| IBIS file stm32h562_563_573_ufbga169.ibs
[IBIS ver] 4.2
[File name] stm32h562_563_573_ufbga169.ibs
[File Rev] 1.1
[Date] 07-05-2024
[Source] Data Created at STMicroelectronics
[Notes]  File originated from ELDO simulations.
[Disclaimer]  This information is for modeling purpose only and is
   not guaranteed. The information is subject to change without
   notice.
[Copyright] Copyright 2024 STMicroelectronics Inc.
|   Component stm32h562_563_573_ufbga169
[Component] stm32h562_563_573_ufbga169
[Manufacturer] STMicroelectronics
[Package]
| variable   typ   min   max
R_pkg  0  NA  NA
L_pkg  0  NA  NA
C_pkg  0  NA  NA
[Pin]   signal_name   model_name
A1  PE2  io8_ft_i3c_spi
A2  PI7  io8_ft_i3c_spi
A3  VDD  power
A4  PB9  io8_ft_i3c_spi
A5  PB6  io8_ft_i3c_spi
A6  PB4  io8_ft_i3c_spi
A7  VDDIO2  power
A8  PG10  io8_ft_i3c_spi
A9  PD3  io8_ft_i3c_spi
A10  VDD  power
A11  PC11  io8_ft_i3c_spi
A12  PA14  io8_ft_i3c_spi
A13  PI2  io8_ft_i3c_spi
B1  PC14-OSC32_IN  io8_ft_i3c_spi
B2  PE3  io8_ft_i3c_spi
B3  VSS  gnd
B4  VCAP  nc
B5  BOOT0  vpphv
B6  PG15  io8_ft_i3c_spi
B7  VSS  gnd
B8  PD7  io8_ft_i3c_spi
B9  PC12  io8_ft_i3c_spi
B10  VSS  gnd
B11  PA15  io8_ft_i3c_spi
B12  PI1  io8_ft_i3c_spi
B13  PI0  io8_ft_i3c_spi
C1  PC15-OSC32_OUT  io8_ft_i3c_spi
C2  PE5  io8_ft_i3c_spi
C3  PI6  io8_ft_i3c_spi
C4  PI4  io8_ft_i3c_spi
C5  PE0  io8_ft_i3c_spi
C6  PB5  io8_ft_i3c_spi
C7  PG14  io8_ft_i3c_spi
C8  PG12  io8_ft_i3c_spi
C9  PD2  io8_ft_i3c_spi
C10  PC10  io8_ft_i3c_spi
C11  PI3  io8_ft_i3c_spi
C12  VSS  gnd
C13  VDD  power
D1  VDD  power
D2  VSS  gnd
D3  PE6  io8_ft_i3c_spi
D4  PE4  io8_ft_i3c_spi
D5  PE1  io8_ft_i3c_spi
D6  PB7  io8_ft_i3c_spi
D7  PG13  io8_ft_i3c_spi
D8  PD5  io8_ft_i3c_spi
D9  PD0  io8_ft_i3c_spi
D10  PH14  io8_ft_i3c_spi
D11  PH15  io8_ft_i3c_spi
D12  PH13  io8_ft_i3c_spi
D13  VDDUSB  power
E1  PF1  io8_ft_i3c_spi
E2  VBAT  power
E3  PI8  io8_ft_i3c_spi
E4  PC13  io8_ft_i3c_spi
E5  PB8  io8_ft_i3c_spi
E6  PB3  io8_ft_i3c_spi
E7  PG11  io8_ft_i3c_spi
E8  PD6  io8_ft_i3c_spi
E9  PD1  io8_ft_i3c_spi
E10  PA10  io8_ft_i3c_spi
E11  PA9  io8_ft_i3c_spi
E12  PA13  io8_ft_i3c_spi
E13  PA12  io8usb_ft_i3c_spi_phy
F1  PF4  io8_ft_i3c_spi
F2  PF2  io8_ft_i3c_spi
F3  PF0  io8_ft_i3c_spi
F4  PI11  io8_ft_i3c_spi
F5  PF3  io8_ft_i3c_spi
F6  PF5  io8_ft_i3c_spi
F7  PG9  io8_ft_i3c_spi
F8  PD4  io8_ft_i3c_spi
F9  PC6  io8_ft_i3c_spi
F10  PC7  io8_ft_i3c_spi
F11  PG8  io8_ft_i3c_spi
F12  PA8  io8_ft_i3c_spi
F13  PA11  io8usb_ft_i3c_spi_phy
G1  VDD  power
G2  VSS  gnd
G3  PF7  io8_ft_i3c_spi
G4  PF6  io8_ft_i3c_spi
G5  PF8  io8_ft_i3c_spi
G6  PF10  io8_ft_i3c_spi
G7  PE8  io8_ft_i3c_spi
G8  PG7  io8_ft_i3c_spi
G9  PG3  io8_ft_i3c_spi
G10  PG5  io8_ft_i3c_spi
G11  PG6  io8_ft_i3c_spi
G12  PC8  io8_ft_i3c_spi
G13  PC9  io8_ft_i3c_spi
H1  PH0-OSC_IN  io8_ft_i3c_spi
H2  PH1-OSC_OUT  io8_ft_i3c_spi
H3  PF9  io8_ft_i3c_spi
H4  NRST  ioreset_ft_v33
H5  PC3  io8_ft_spi
H6  PC5  io8_ft_spi
H7  PF13  io8_ft_spi
H8  PE10  io8_ft_i3c_spi
H9  PD15  io8_ft_i3c_spi
H10  PD11  io8_ft_i3c_spi
H11  PD14  io8_ft_i3c_spi
H12  VSS  gnd
H13  VDD  power
J1  PC0  io8_ft_spi
J2  PC1  io8_ft_spi
J3  PC2  io8_ft_spi
J4  PA0  io8_ft_spi
J5  PA1  io8_ft_spi_tamp
J6  PF11  io8_ft_spi
J7  PF15  io8_ft_i3c_spi
J8  PE14  io8_ft_i3c_spi
J9  PD9  io8_ft_i3c_spi
J10  PB15  io8_ft_spi
J11  PD10  io8_ft_i3c_spi
J12  PG2  io8_ft_i3c_spi
J13  PG4  io8_ft_i3c_spi
K1  VREFM  nc
K2  VSSA  nc
K3  PH2  io8_ft_i3c_spi
K4  PA5  io8_ft_spi
K5  PA7  io8_ft_spi
K6  PB1  io8_ft_spi
K7  PG1  io8_ft_i3c_spi
K8  PE12  io8_ft_i3c_spi
K9  PB10  io8_ft_i3c_spi
K10  PH6  io8_ft_i3c_spi
K11  PB12  io8_ft_i3c_spi
K12  PD12  io8_ft_i3c_spi
K13  PD13  io8_ft_i3c_spi
L1  VDDA  nc
L2  VREFP  nc
L3  PA2  io8_ft_spi
L4  PA4  io8_ft_spi
L5  PB0  io8_ft_spi
L6  PB2  io8_ft_i3c_spi
L7  PG0  io8_ft_i3c_spi
L8  PE9  io8_ft_i3c_spi
L9  PE13  io8_ft_i3c_spi
L10  PH7  io8_ft_i3c_spi
|L11  PB13  io8usb_ft_pd
L11  PB13  nc
L12  PD8  io8_ft_i3c_spi
L13  VDD  power
M1  VDD  power
M2  VSS  gnd
M3  PH5  io8_ft_i3c_spi
M4  VSS  gnd
M5  PA6  io8_ft_spi
M6  PF14  io8_ft_spi
M7  VSS  gnd
M8  PE11  io8_ft_i3c_spi
M9  PB11  io8_ft_i3c_spi
M10  PH8  io8_ft_i3c_spi
M11  PH10  io8_ft_i3c_spi
M12  VSS  gnd
|M13  PB14  io8usb_ft_pd
M13  PB14  nc
N1  PH4  io8_ft_i3c_spi
N2  PH3  io8_ft_i3c_spi
N3  PA3  io8_ft_spi
N4  VDD  power
N5  PC4  io8_ft_spi
N6  PF12  io8_ft_spi
N7  VDD  power
N8  PE7  io8_ft_i3c_spi
N9  PE15  io8_ft_i3c_spi
N10  VCAP  nc
N11  VDD  power
N12  PH11  io8_ft_i3c_spi
N13  PH12  io8_ft_i3c_spi
[Package Model]   484-ufbga-7x7-169-ldo-221014
[Pin Mapping]   pulldown_ref   pullup_ref   | Comment
A1  gndio  vddiom
A2  gndio  vddiom
A3  nc  vddiom
A4  gndio  vddiom  | Depending on IO usage
| A4  gndio  vddmmc  | Depending on IO usage
A5  gndio  vddiom  | Depending on IO usage
| A5  gndio  vddmmc  | Depending on IO usage
A6  gndio  vddiom  | Depending on IO usage
| A6  gndio  vddmmc  | Depending on IO usage
A7  nc  vddmmc
A8  gndio  vddiom  | Depending on IO usage
| A8  gndio  vddmmc  | Depending on IO usage
A9  gndio  vddiom
A10  nc  vddiom
A11  gndio  vddiom
A12  gndio  vddiom
A13  gndio  vddiom
B1  gndio  vddiom  | Depending on IO usage
| B1  gndio  vsw  | Depending on IO usage
B2  gndio  vddiom
B3  gndio  nc
B4  nc  nc
B5  gndio  vddiom  | Depending on IO usage
| B5  gndio  vddmmc  | Depending on IO usage
B6  gndio  vddiom  | Depending on IO usage
| B6  gndio  vddmmc  | Depending on IO usage
B7  gndio  nc
B8  gndio  vddiom  | Depending on IO usage
| B8  gndio  vddmmc  | Depending on IO usage
B9  gndio  vddiom
B10  gndio  nc
B11  gndio  vddiom
B12  gndio  vddiom
B13  gndio  vddiom
C1  gndio  vddiom  | Depending on IO usage
| C1  gndio  vsw  | Depending on IO usage
C2  gndio  vddiom
C3  gndio  vddiom
C4  gndio  vddiom
C5  gndio  vddiom  | Depending on IO usage
| C5  gndio  vddmmc  | Depending on IO usage
C6  gndio  vddiom  | Depending on IO usage
| C6  gndio  vddmmc  | Depending on IO usage
C7  gndio  vddiom  | Depending on IO usage
| C7  gndio  vddmmc  | Depending on IO usage
C8  gndio  vddiom  | Depending on IO usage
| C8  gndio  vddmmc  | Depending on IO usage
C9  gndio  vddiom
C10  gndio  vddiom
C11  gndio  vddiom
C12  gndio  nc
C13  nc  vddiom
D1  nc  vddiom
D2  gndio  nc
D3  gndio  vddiom
D4  gndio  vddiom
D5  gndio  vddiom  | Depending on IO usage
| D5  gndio  vddmmc  | Depending on IO usage
D6  gndio  vddiom  | Depending on IO usage
| D6  gndio  vddmmc  | Depending on IO usage
D7  gndio  vddiom  | Depending on IO usage
| D7  gndio  vddmmc  | Depending on IO usage
D8  gndio  vddiom
D9  gndio  vddiom
D10  gndio  vddiom
D11  gndio  vddiom
D12  gndio  vddiom
D13  nc  vddusb
E1  gndio  vddiom
E2  nc  vsw
E3  gndio  vddiom  | Depending on IO usage
| E3  gndio  vsw  | Depending on IO usage
E4  gndio  vddiom  | Depending on IO usage
| E4  gndio  vsw  | Depending on IO usage
E5  gndio  vddiom  | Depending on IO usage
| E5  gndio  vddmmc  | Depending on IO usage
E6  gndio  vddiom  | Depending on IO usage
| E6  gndio  vddmmc  | Depending on IO usage
E7  gndio  vddiom  | Depending on IO usage
| E7  gndio  vddmmc  | Depending on IO usage
E8  gndio  vddiom  | Depending on IO usage
| E8  gndio  vddmmc  | Depending on IO usage
E9  gndio  vddiom
E10  gndio  vddiom  | Depending on IO usage
| E10  gndio  vddusb  | Depending on IO usage
E11  gndio  vddiom  | Depending on IO usage
| E11  gndio  vddusb  | Depending on IO usage
E12  gndio  vddiom  | Depending on IO usage
| E12  gndio  vddusb  | Depending on IO usage
E13  gndio  vddiom  | Depending on IO usage
| E13  gndio  vddusb  | Depending on IO usage
F1  gndio  vddiom
F2  gndio  vddiom
F3  gndio  vddiom
F4  gndio  vddiom
F5  gndio  vddiom
F6  gndio  vddiom
F7  gndio  vddiom  | Depending on IO usage
| F7  gndio  vddmmc  | Depending on IO usage
F8  gndio  vddiom
F9  gndio  vddiom
F10  gndio  vddiom
F11  gndio  vddiom
F12  gndio  vddiom
F13  gndio  vddiom  | Depending on IO usage
| F13  gndio  vddusb  | Depending on IO usage
G1  nc  vddiom
G2  gndio  nc
G3  gndio  vddiom
G4  gndio  vddiom
G5  gndio  vddiom
G6  gndio  vddiom
G7  gndio  vddiom
G8  gndio  vddiom
G9  gndio  vddiom
G10  gndio  vddiom
G11  gndio  vddiom
G12  gndio  vddiom
G13  gndio  vddiom
H1  gndio  vddiom
H2  gndio  vddiom
H3  gndio  vddiom
H4  gndio  vddiom
H5  gndio  vddiom
H6  gndio  vddiom
H7  gndio  vddiom
H8  gndio  vddiom
H9  gndio  vddiom
H10  gndio  vddiom
H11  gndio  vddiom
H12  gndio  nc
H13  nc  vddiom
J1  gndio  vddiom
J2  gndio  vddiom
J3  gndio  vddiom
J4  gndio  vddiom
J5  gndio  vddiom
J6  gndio  vddiom
J7  gndio  vddiom
J8  gndio  vddiom
J9  gndio  vddiom
J10  gndio  vddiom
J11  gndio  vddiom
J12  gndio  vddiom
J13  gndio  vddiom
K1  nc  nc
K2  nc  nc
K3  gndio  vddiom
K4  gndio  vddiom
K5  gndio  vddiom
K6  gndio  vddiom
K7  gndio  vddiom
K8  gndio  vddiom
K9  gndio  vddiom
K10  gndio  vddiom
K11  gndio  vddiom
K12  gndio  vddiom
K13  gndio  vddiom
L1  nc  nc
L2  nc  nc
L3  gndio  vddiom
L4  gndio  vddiom
L5  gndio  vddiom
L6  gndio  vddiom
L7  gndio  vddiom
L8  gndio  vddiom
L9  gndio  vddiom
L10  gndio  vddiom
|L11  gndio  vddiom
L11  nc nc
L12  gndio  vddiom
L13  nc  vddiom
M1  nc  vddiom
M2  gndio  nc
M3  gndio  vddiom
M4  gndio  nc
M5  gndio  vddiom
M6  gndio  vddiom
M7  gndio  nc
M8  gndio  vddiom
M9  gndio  vddiom
M10  gndio  vddiom
M11  gndio  vddiom
M12  gndio  nc
|M13  gndio  vddiom
M13  nc nc
N1  gndio  vddiom
N2  gndio  vddiom
N3  gndio  vddiom
N4  nc  vddiom
N5  gndio  vddiom
N6  gndio  vddiom
N7  nc  vddiom
N8  gndio  vddiom
N9  gndio  vddiom
N10  nc  nc
N11  nc  vddiom
N12  gndio  vddiom
N13  gndio  vddiom
[Model Selector] io8_ft_i3c_spi
io8_ft_spi_ls_1v2 "io8_ft spi low speed @ 1.2V"
io8_ft_spi_ls_1v8 "io8_ft spi low speed @ 1.8V"
io8_ft_spi_ls_3v3 "io8_ft spi low speed @ 3.3V"
io8_ft_spi_ms_1v2 "io8_ft spi med speed @ 1.2V"
io8_ft_spi_ms_1v8 "io8_ft spi med speed @ 1.8V"
io8_ft_spi_ms_3v3 "io8_ft spi med speed @ 3.3V"
io8_ft_spi_fs_1v2 "io8_ft spi fast speed @ 1.2V"
io8_ft_spi_fs_1v8 "io8_ft spi fast speed @ 1.8V"
io8_ft_spi_fs_3v3 "io8_ft spi fast speed @ 3.3V"
io8_ft_spi_hs_1v2 "io8_ft spi high speed @ 1.2V"
io8_ft_spi_hs_1v8 "io8_ft spi high speed @ 1.8V"
io8_ft_spi_hs_3v3 "io8_ft spi high speed @ 3.3V"
io8_ft_hslv_spi_ls_1v2 "io8_ft spi hslv low speed @ 1.2V"
io8_ft_hslv_spi_ls_1v8 "io8_ft spi hslv low speed @ 1.8V"
io8_ft_hslv_spi_ls_2v5 "io8_ft spi hslv low speed @ 2.5V"
io8_ft_hslv_spi_ms_1v2 "io8_ft spi hslv med speed @ 1.2V"
io8_ft_hslv_spi_ms_1v8 "io8_ft spi hslv med speed @ 1.8V"
io8_ft_hslv_spi_ms_2v5 "io8_ft spi hslv med speed @ 2.5V"
io8_ft_hslv_spi_fs_1v2 "io8_ft spi hslv fast speed @ 1.2V"
io8_ft_hslv_spi_fs_1v8 "io8_ft spi hslv fast speed @ 1.8V"
io8_ft_hslv_spi_fs_2v5 "io8_ft spi hslv fast speed @ 2.5V"
io8_ft_hslv_spi_hs_1v2 "io8_ft spi hslv high speed @ 1.2V"
io8_ft_hslv_spi_hs_1v8 "io8_ft spi hslv high speed @ 1.8V"
io8_ft_hslv_spi_hs_2v5 "io8_ft spi hslv high speed @ 2.5V"
io8_ft_i3c_spi_ls_1v2 "io8_ft i3c spi open-drain low speed @ 1.2V"
io8_ft_i3c_spi_ls_1v8 "io8_ft i3c spi open-drain low speed @ 1.8V"
io8_ft_i3c_spi_ls_3v3 "io8_ft i3c spi open-drain low speed @ 3.3V"
io8_ft_i3c_spi_ms_1v2 "io8_ft i3c spi open-drain med speed @ 1.2V"
io8_ft_i3c_spi_ms_1v8 "io8_ft i3c spi open-drain med speed @ 1.8V"
io8_ft_i3c_spi_ms_3v3 "io8_ft i3c spi open-drain med speed @ 3.3V"
io8_ft_i3c_spi_fs_1v2 "io8_ft i3c spi open-drain fast speed @ 1.2V"
io8_ft_i3c_spi_fs_1v8 "io8_ft i3c spi open-drain fast speed @ 1.8V"
io8_ft_i3c_spi_fs_3v3 "io8_ft i3c spi open-drain fast speed @ 3.3V"
io8_ft_i3c_spi_hs_1v2 "io8_ft i3c spi open-drain high speed @ 1.2V"
io8_ft_i3c_spi_hs_1v8 "io8_ft i3c spi open-drain high speed @ 1.8V"
io8_ft_i3c_spi_hs_3v3 "io8_ft i3c spi open-drain high speed @ 3.3V"
io8_ft_hslv_i3c_spi_ls_1v2 "io8_ft hslv i3c spi open-drain low speed @ 1.2V"
io8_ft_hslv_i3c_spi_ls_1v8 "io8_ft hslv i3c spi open-drain low speed @ 1.8V"
io8_ft_hslv_i3c_spi_ls_2v5 "io8_ft hslv i3c spi open-drain low speed @ 2.5V"
io8_ft_hslv_i3c_spi_ms_1v2 "io8_ft hslv i3c spi open-drain med speed @ 1.2V"
io8_ft_hslv_i3c_spi_ms_1v8 "io8_ft hslv i3c spi open-drain med speed @ 1.8V"
io8_ft_hslv_i3c_spi_ms_2v5 "io8_ft hslv i3c spi open-drain med speed @ 2.5V"
io8_ft_hslv_i3c_spi_fs_1v2 "io8_ft hslv i3c spi open-drain fast speed @ 1.2V"
io8_ft_hslv_i3c_spi_fs_1v8 "io8_ft hslv i3c spi open-drain fast speed @ 1.8V"
io8_ft_hslv_i3c_spi_fs_2v5 "io8_ft hslv i3c spi open-drain fast speed @ 2.5V"
io8_ft_hslv_i3c_spi_hs_1v2 "io8_ft hslv i3c spi open-drain high speed @ 1.2V"
io8_ft_hslv_i3c_spi_hs_1v8 "io8_ft hslv i3c spi open-drain high speed @ 1.8V"
io8_ft_hslv_i3c_spi_hs_2v5 "io8_ft hslv i3c spi open-drain high speed @ 2.5V"
io8_ft_i3c_fmp_spi_3v3 "io8_ft i3c fm+ spi open-drain @ 3.3V"
io8_ft_i3c_fmp_spi_1v8 "io8_ft i3c fm+ spi open-drain @ 1.8V"
io8_ft_i3c_fmp_spi_1v2 "io8_ft i3c fm+ spi open-drain @ 1.2V"
[Model Selector] io8_ft_spi
io8_ft_spi_ls_1v2 "io8_ft spi low speed @ 1.2V"
io8_ft_spi_ls_1v8 "io8_ft spi low speed @ 1.8V"
io8_ft_spi_ls_3v3 "io8_ft spi low speed @ 3.3V"
io8_ft_spi_ms_1v2 "io8_ft spi med speed @ 1.2V"
io8_ft_spi_ms_1v8 "io8_ft spi med speed @ 1.8V"
io8_ft_spi_ms_3v3 "io8_ft spi med speed @ 3.3V"
io8_ft_spi_fs_1v2 "io8_ft spi fast speed @ 1.2V"
io8_ft_spi_fs_1v8 "io8_ft spi fast speed @ 1.8V"
io8_ft_spi_fs_3v3 "io8_ft spi fast speed @ 3.3V"
io8_ft_spi_hs_1v2 "io8_ft spi high speed @ 1.2V"
io8_ft_spi_hs_1v8 "io8_ft spi high speed @ 1.8V"
io8_ft_spi_hs_3v3 "io8_ft spi high speed @ 3.3V"
io8_ft_hslv_spi_ls_1v2 "io8_ft spi hslv low speed @ 1.2V"
io8_ft_hslv_spi_ls_1v8 "io8_ft spi hslv low speed @ 1.8V"
io8_ft_hslv_spi_ls_2v5 "io8_ft spi hslv low speed @ 2.5V"
io8_ft_hslv_spi_ms_1v2 "io8_ft spi hslv med speed @ 1.2V"
io8_ft_hslv_spi_ms_1v8 "io8_ft spi hslv med speed @ 1.8V"
io8_ft_hslv_spi_ms_2v5 "io8_ft spi hslv med speed @ 2.5V"
io8_ft_hslv_spi_fs_1v2 "io8_ft spi hslv fast speed @ 1.2V"
io8_ft_hslv_spi_fs_1v8 "io8_ft spi hslv fast speed @ 1.8V"
io8_ft_hslv_spi_fs_2v5 "io8_ft spi hslv fast speed @ 2.5V"
io8_ft_hslv_spi_hs_1v2 "io8_ft spi hslv high speed @ 1.2V"
io8_ft_hslv_spi_hs_1v8 "io8_ft spi hslv high speed @ 1.8V"
io8_ft_hslv_spi_hs_2v5 "io8_ft spi hslv high speed @ 2.5V"
[Model Selector] io8_ft_spi_tamp
io8_ft_spi_ls_1v2 "io8_ft spi low speed @ 1.2V"
io8_ft_spi_ls_1v8 "io8_ft spi low speed @ 1.8V"
io8_ft_spi_ls_3v3 "io8_ft spi low speed @ 3.3V"
io8_ft_spi_ms_1v2 "io8_ft spi med speed @ 1.2V"
io8_ft_spi_ms_1v8 "io8_ft spi med speed @ 1.8V"
io8_ft_spi_ms_3v3 "io8_ft spi med speed @ 3.3V"
io8_ft_spi_fs_1v2 "io8_ft spi fast speed @ 1.2V"
io8_ft_spi_fs_1v8 "io8_ft spi fast speed @ 1.8V"
io8_ft_spi_fs_3v3 "io8_ft spi fast speed @ 3.3V"
io8_ft_spi_hs_1v2 "io8_ft spi high speed @ 1.2V"
io8_ft_spi_hs_1v8 "io8_ft spi high speed @ 1.8V"
io8_ft_spi_hs_3v3 "io8_ft spi high speed @ 3.3V"
io8_ft_hslv_spi_ls_1v2 "io8_ft spi hslv low speed @ 1.2V"
io8_ft_hslv_spi_ls_1v8 "io8_ft spi hslv low speed @ 1.8V"
io8_ft_hslv_spi_ls_2v5 "io8_ft spi hslv low speed @ 2.5V"
io8_ft_hslv_spi_ms_1v2 "io8_ft spi hslv med speed @ 1.2V"
io8_ft_hslv_spi_ms_1v8 "io8_ft spi hslv med speed @ 1.8V"
io8_ft_hslv_spi_ms_2v5 "io8_ft spi hslv med speed @ 2.5V"
io8_ft_hslv_spi_fs_1v2 "io8_ft spi hslv fast speed @ 1.2V"
io8_ft_hslv_spi_fs_1v8 "io8_ft spi hslv fast speed @ 1.8V"
io8_ft_hslv_spi_fs_2v5 "io8_ft spi hslv fast speed @ 2.5V"
io8_ft_hslv_spi_hs_1v2 "io8_ft spi hslv high speed @ 1.2V"
io8_ft_hslv_spi_hs_1v8 "io8_ft spi hslv high speed @ 1.8V"
io8_ft_hslv_spi_hs_2v5 "io8_ft spi hslv high speed @ 2.5V"
io8_ft_tamp_v33_1v2 "io8_ft tamp V33 @ 1.2V"
io8_ft_tamp_v33_1v8 "io8_ft tamp V33 @ 1.2V"
io8_ft_tamp_v33_3v3 "io8_ft tamp V33 @ 1.2V"
[Model Selector] io8usb_ft_i3c_spi_phy
io8_ft_spi_ls_1v2 "io8_ft spi low speed @ 1.2V"
io8_ft_spi_ls_1v8 "io8_ft spi low speed @ 1.8V"
io8_ft_spi_ls_3v3 "io8_ft spi low speed @ 3.3V"
io8_ft_spi_ms_1v2 "io8_ft spi med speed @ 1.2V"
io8_ft_spi_ms_1v8 "io8_ft spi med speed @ 1.8V"
io8_ft_spi_ms_3v3 "io8_ft spi med speed @ 3.3V"
io8_ft_spi_fs_1v2 "io8_ft spi fast speed @ 1.2V"
io8_ft_spi_fs_1v8 "io8_ft spi fast speed @ 1.8V"
io8_ft_spi_fs_3v3 "io8_ft spi fast speed @ 3.3V"
io8_ft_spi_hs_1v2 "io8_ft spi high speed @ 1.2V"
io8_ft_spi_hs_1v8 "io8_ft spi high speed @ 1.8V"
io8_ft_spi_hs_3v3 "io8_ft spi high speed @ 3.3V"
io8_ft_hslv_spi_ls_1v2 "io8_ft spi hslv low speed @ 1.2V"
io8_ft_hslv_spi_ls_1v8 "io8_ft spi hslv low speed @ 1.8V"
io8_ft_hslv_spi_ls_2v5 "io8_ft spi hslv low speed @ 2.5V"
io8_ft_hslv_spi_ms_1v2 "io8_ft spi hslv med speed @ 1.2V"
io8_ft_hslv_spi_ms_1v8 "io8_ft spi hslv med speed @ 1.8V"
io8_ft_hslv_spi_ms_2v5 "io8_ft spi hslv med speed @ 2.5V"
io8_ft_hslv_spi_fs_1v2 "io8_ft spi hslv fast speed @ 1.2V"
io8_ft_hslv_spi_fs_1v8 "io8_ft spi hslv fast speed @ 1.8V"
io8_ft_hslv_spi_fs_2v5 "io8_ft spi hslv fast speed @ 2.5V"
io8_ft_hslv_spi_hs_1v2 "io8_ft spi hslv high speed @ 1.2V"
io8_ft_hslv_spi_hs_1v8 "io8_ft spi hslv high speed @ 1.8V"
io8_ft_hslv_spi_hs_2v5 "io8_ft spi hslv high speed @ 2.5V"
io8_ft_i3c_spi_ls_1v2 "io8_ft i3c spi open-drain low speed @ 1.2V"
io8_ft_i3c_spi_ls_1v8 "io8_ft i3c spi open-drain low speed @ 1.8V"
io8_ft_i3c_spi_ls_3v3 "io8_ft i3c spi open-drain low speed @ 3.3V"
io8_ft_i3c_spi_ms_1v2 "io8_ft i3c spi open-drain med speed @ 1.2V"
io8_ft_i3c_spi_ms_1v8 "io8_ft i3c spi open-drain med speed @ 1.8V"
io8_ft_i3c_spi_ms_3v3 "io8_ft i3c spi open-drain med speed @ 3.3V"
io8_ft_i3c_spi_fs_1v2 "io8_ft i3c spi open-drain fast speed @ 1.2V"
io8_ft_i3c_spi_fs_1v8 "io8_ft i3c spi open-drain fast speed @ 1.8V"
io8_ft_i3c_spi_fs_3v3 "io8_ft i3c spi open-drain fast speed @ 3.3V"
io8_ft_i3c_spi_hs_1v2 "io8_ft i3c spi open-drain high speed @ 1.2V"
io8_ft_i3c_spi_hs_1v8 "io8_ft i3c spi open-drain high speed @ 1.8V"
io8_ft_i3c_spi_hs_3v3 "io8_ft i3c spi open-drain high speed @ 3.3V"
io8_ft_hslv_i3c_spi_ls_1v2 "io8_ft hslv i3c spi open-drain low speed @ 1.2V"
io8_ft_hslv_i3c_spi_ls_1v8 "io8_ft hslv i3c spi open-drain low speed @ 1.8V"
io8_ft_hslv_i3c_spi_ls_2v5 "io8_ft hslv i3c spi open-drain low speed @ 2.5V"
io8_ft_hslv_i3c_spi_ms_1v2 "io8_ft hslv i3c spi open-drain med speed @ 1.2V"
io8_ft_hslv_i3c_spi_ms_1v8 "io8_ft hslv i3c spi open-drain med speed @ 1.8V"
io8_ft_hslv_i3c_spi_ms_2v5 "io8_ft hslv i3c spi open-drain med speed @ 2.5V"
io8_ft_hslv_i3c_spi_fs_1v2 "io8_ft hslv i3c spi open-drain fast speed @ 1.2V"
io8_ft_hslv_i3c_spi_fs_1v8 "io8_ft hslv i3c spi open-drain fast speed @ 1.8V"
io8_ft_hslv_i3c_spi_fs_2v5 "io8_ft hslv i3c spi open-drain fast speed @ 2.5V"
io8_ft_hslv_i3c_spi_hs_1v2 "io8_ft hslv i3c spi open-drain high speed @ 1.2V"
io8_ft_hslv_i3c_spi_hs_1v8 "io8_ft hslv i3c spi open-drain high speed @ 1.8V"
io8_ft_hslv_i3c_spi_hs_2v5 "io8_ft hslv i3c spi open-drain high speed @ 2.5V"
io8_ft_i3c_fmp_spi_3v3 "io8_ft i3c fm+ spi open-drain @ 3.3V"
io8_ft_i3c_fmp_spi_1v8 "io8_ft i3c fm+ spi open-drain @ 1.8V"
io8_ft_i3c_fmp_spi_1v2 "io8_ft i3c fm+ spi open-drain @ 1.2V"
io8usb_ft_phy_ls_2v5 "iousb ft low speed @ 2.5V"
io8usb_ft_phy_ls_3v3 "iousb ft low speed @ 3.3V"
io8usb_ft_phy_fs_2v5 "iousb ft fast speed @ 2.5V"
io8usb_ft_phy_fs_3v3 "iousb ft fast speed @ 3.3V"
[Model Selector] ioreset_ft_v33
ioreset_ft_v33_1v2 "Reset PAD. 5V tolerant. 1.2V range"
ioreset_ft_v33_1v8 "Reset PAD. 5V tolerant. 1.8V range"
ioreset_ft_v33_3v3 "Reset PAD. 5V tolerant. 3.3V range"
[Model Selector] vpphv
vpphv_1v2 "Flash Test cell v33 = 1.2 V range"
vpphv_1v8 "Flash Test cell v33 = 1.8 V range"
vpphv_3v3 "Flash Test cell v33 = 3.3 V range"
[Define Package Model]  484-ufbga-7x7-169-ldo-221014
[Manufacturer]  unknown
[OEM]  unknown
[Description]  unknown
[Number Of Pins]  149
[Pin Numbers]
| Pin Name Terminal   Net Name   Starting Node   Ending Node
B5 | BOOT0
H4 | NRST
J4 | PA0
J5 | PA1
L3 | PA2
N3 | PA3
L4 | PA4
K4 | PA5
M5 | PA6
K5 | PA7
F12 | PA8
E11 | PA9
E10 | PA10
F13 | PA11
E13 | PA12
E12 | PA13
A12 | PA14
B11 | PA15
L5 | PB0
K6 | PB1
L6 | PB2
E6 | PB3
A6 | PB4
C6 | PB5
A5 | PB6
D6 | PB7
E5 | PB8
A4 | PB9
K9 | PB10
M9 | PB11
K11 | PB12
L11 | PB13
M13 | PB14
J10 | PB15
J1 | PC0
J2 | PC1
J3 | PC2
H5 | PC3
N5 | PC4
H6 | PC5
F9 | PC6
F10 | PC7
G12 | PC8
G13 | PC9
C10 | PC10
A11 | PC11
B9 | PC12
E4 | PC13
B1 | PC14-OSC32_IN
C1 | PC15-OSC32_OUT
D9 | PD0
E9 | PD1
C9 | PD2
A9 | PD3
F8 | PD4
D8 | PD5
E8 | PD6
B8 | PD7
L12 | PD8
J9 | PD9
J11 | PD10
H10 | PD11
K12 | PD12
K13 | PD13
H11 | PD14
H9 | PD15
C5 | PE0
D5 | PE1
A1 | PE2
B2 | PE3
D4 | PE4
C2 | PE5
D3 | PE6
N8 | PE7
G7 | PE8
L8 | PE9
H8 | PE10
M8 | PE11
K8 | PE12
L9 | PE13
J8 | PE14
N9 | PE15
F3 | PF0
E1 | PF1
F2 | PF2
F5 | PF3
F1 | PF4
F6 | PF5
G4 | PF6
G3 | PF7
G5 | PF8
H3 | PF9
G6 | PF10
J6 | PF11
N6 | PF12
H7 | PF13
M6 | PF14
J7 | PF15
L7 | PG0
K7 | PG1
J12 | PG2
G9 | PG3
J13 | PG4
G10 | PG5
G11 | PG6
G8 | PG7
F11 | PG8
F7 | PG9
A8 | PG10
E7 | PG11
C8 | PG12
D7 | PG13
C7 | PG14
B6 | PG15
H1 | PH0-OSC_IN
H2 | PH1-OSC_OUT
K3 | PH2
N2 | PH3
N1 | PH4
M3 | PH5
K10 | PH6
L10 | PH7
M10 | PH8
M11 | PH10
N12 | PH11
N13 | PH12
D12 | PH13
D10 | PH14
D11 | PH15
B13 | PI0
B12 | PI1
A13 | PI2
C11 | PI3
C4 | PI4
C3 | PI6
A2 | PI7
E3 | PI8
F4 | PI11
E2 | VBAT
N10 | VCAP
B4 | VCAP
D13 | VDDUSB
A3 | VDD
L1 | VDDA
A7 | VDDIO2
K1 | VREFM
L2 | VREFP
B3 | VSS
K2 | VSSA
|[Merged Pins]  A3
|A10  |  VDD
|C13  |  VDD
|D1  |  VDD
|G1  |  VDD
|H13  |  VDD
|L13  |  VDD
|M1  |  VDD
|N4  |  VDD
|N7  |  VDD
|N11  |  VDD
|[Merged Pins]  B3
|B7  |  VSS
|B10  |  VSS
|C12  |  VSS
|D2  |  VSS
|G2  |  VSS
|H12  |  VSS
|M2  |  VSS
|M4  |  VSS
|M7  |  VSS
|M12  |  VSS
[Model Data]
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[End Model Data]
[End Package Model]
|End [Component]
| Models and submodels in the file (64): io8_ft_hslv_i3c_spi_fs_1v2 (I/O_open_drain), io8_ft_hslv_i3c_spi_fs_1v8 (I/O_open_drain), io8_ft_hslv_i3c_spi_fs_2v5 (I/O_open_drain), io8_ft_hslv_i3c_spi_hs_1v2 (I/O_open_drain), io8_ft_hslv_i3c_spi_hs_1v8 (I/O_open_drain), io8_ft_hslv_i3c_spi_hs_2v5 (I/O_open_drain), io8_ft_hslv_i3c_spi_ls_1v2 (I/O_open_drain), io8_ft_hslv_i3c_spi_ls_1v8 (I/O_open_drain), io8_ft_hslv_i3c_spi_ls_2v5 (I/O_open_drain), io8_ft_hslv_i3c_spi_ms_1v2 (I/O_open_drain), io8_ft_hslv_i3c_spi_ms_1v8 (I/O_open_drain), io8_ft_hslv_i3c_spi_ms_2v5 (I/O_open_drain), io8_ft_hslv_spi_fs_1v2 (I/O), io8_ft_hslv_spi_fs_1v8 (I/O), io8_ft_hslv_spi_fs_2v5 (I/O), io8_ft_hslv_spi_hs_1v2 (I/O), io8_ft_hslv_spi_hs_1v8 (I/O), io8_ft_hslv_spi_hs_2v5 (I/O), io8_ft_hslv_spi_ls_1v2 (I/O), io8_ft_hslv_spi_ls_1v8 (I/O), io8_ft_hslv_spi_ls_2v5 (I/O), io8_ft_hslv_spi_ms_1v2 (I/O), io8_ft_hslv_spi_ms_1v8 (I/O), io8_ft_hslv_spi_ms_2v5 (I/O), io8_ft_i3c_fmp_spi_1v2 (I/O_open_drain), io8_ft_i3c_fmp_spi_1v8 (I/O_open_drain), io8_ft_i3c_fmp_spi_3v3 (I/O_open_drain), io8_ft_i3c_spi_fs_1v2 (I/O_open_drain), io8_ft_i3c_spi_fs_1v8 (I/O_open_drain), io8_ft_i3c_spi_fs_3v3 (I/O_open_drain), io8_ft_i3c_spi_hs_1v2 (I/O_open_drain), io8_ft_i3c_spi_hs_1v8 (I/O_open_drain), io8_ft_i3c_spi_hs_3v3 (I/O_open_drain), io8_ft_i3c_spi_ls_1v2 (I/O_open_drain), io8_ft_i3c_spi_ls_1v8 (I/O_open_drain), io8_ft_i3c_spi_ls_3v3 (I/O_open_drain), io8_ft_i3c_spi_ms_1v2 (I/O_open_drain), io8_ft_i3c_spi_ms_1v8 (I/O_open_drain), io8_ft_i3c_spi_ms_3v3 (I/O_open_drain), io8_ft_spi_fs_1v2 (I/O), io8_ft_spi_fs_1v8 (I/O), io8_ft_spi_fs_3v3 (I/O), io8_ft_spi_hs_1v2 (I/O), io8_ft_spi_hs_1v8 (I/O), io8_ft_spi_hs_3v3 (I/O), io8_ft_spi_ls_1v2 (I/O), io8_ft_spi_ls_1v8 (I/O), io8_ft_spi_ls_3v3 (I/O), io8_ft_spi_ms_1v2 (I/O), io8_ft_spi_ms_1v8 (I/O), io8_ft_spi_ms_3v3 (I/O), io8_ft_tamp_v33_1v2 (I/O), io8_ft_tamp_v33_1v8 (I/O), io8_ft_tamp_v33_3v3 (I/O), io8usb_ft_phy_fs_2v5 (I/O), io8usb_ft_phy_fs_3v3 (I/O), io8usb_ft_phy_ls_2v5 (I/O), io8usb_ft_phy_ls_3v3 (I/O), ioreset_ft_v33_1v2 (I/O_open_drain), ioreset_ft_v33_1v8 (I/O_open_drain), ioreset_ft_v33_3v3 (I/O_open_drain), vpphv_1v2 (Input), vpphv_1v8 (Input), vpphv_3v3 (Input)
